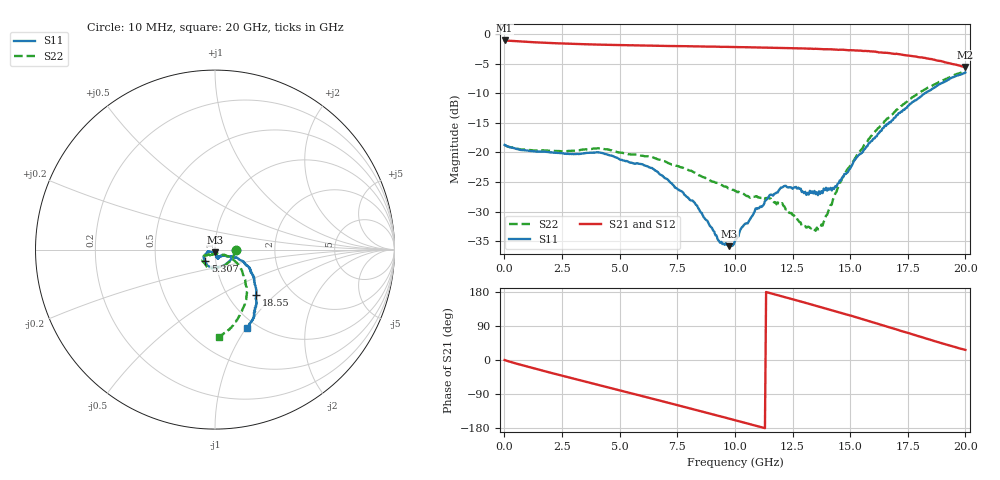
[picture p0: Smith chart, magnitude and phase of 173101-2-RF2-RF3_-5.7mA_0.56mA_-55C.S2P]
!  2-Port S-parameters saved by WinCal
! VAR MeasName=S-Parameters (CALIBRATED_DATA) read from VNA (N5242A)
! VAR MeasDate=2017-7-20 10:24:18
! VAR NAME=173101-2-RF2-RF3_-5.7mA_0.56mA_-55C
! VAR FILENAME=173101-2-RF2-RF3_-5.7mA_0.56mA_-55C.S2P
! VAR DATE=2017-7-20 10:24:18
! VAR PHYS_PORTS=1,2
# Hz S DB R 50
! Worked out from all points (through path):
!   401 points, 10 MHz to 20 GHz, reference 50 ohm
!   highest |S21| = -1.10 dB at 10 MHz (marker M1); lowest = -5.6 dB at 20 GHz (marker M2)
!   group delay of S21, straight-line fit = 45.8 ps
!   lowest |S11| = -35.8 dB at 9.755 GHz (marker M3), VSWR 1.03, Z = 50 - j1.61 ohm
!   |S11| at or under -10 dB: start of sweep to 18.25 GHz
!   |S22| runs from -33.2 to -6.3 dB; largest |S21 - S12| = 0.0092
!   S11 on the Smith chart (normalised r, x): 10 MHz: 1.26, -0.01; 5.307 GHz: 0.89, -0.12; 18.55 GHz: 1.34, -0.77; 20 GHz: 0.90, -1.01
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1e7  -18.75 -2.0  -1.10 -0.0  -1.11 -0.1  -18.75 -1.9
1.559225e9  -19.88 -55.0  -1.46 -26.5  -1.47 -26.6  -19.68 -55.0
3.358325e9  -20.22 -97.9  -1.72 -54.7  -1.73 -54.8  -19.55 -96.1
4.157925e9  -20.05 -113.5  -1.81 -67.1  -1.83 -67.1  -19.32 -111.3
5.30735e9  -21.46 -129.9  -1.91 -84.8  -1.93 -84.8  -20.22 -124.7
6.70665e9  -23.56 -150.4  -2.00 -106.7  -2.00 -106.6  -21.23 -141.5
8.255875e9  -28.53 -163.2  -2.12 -130.9  -2.13 -130.9  -23.42 -151.2
9.355325e9  -35.25 -117.4  -2.18 -148.5  -2.18 -148.4  -25.41 -144.9
9.755125e9  -35.84 -89.0  -2.20 -154.8  -2.20 -154.9  -26.07 -145.6
1.0005e10  -34.94 -84.9  -2.21 -158.8  -2.23 -158.9  -26.49 -144.8
1.090455e10  -29.45 -74.0  -2.28 -173.3  -2.30 -173.3  -27.43 -130.9
1.205398e10  -25.93 -74.3  -2.37 167.9  -2.38 167.9  -28.59 -123.0
1.30035e10  -26.90 -59.4  -2.46 151.9  -2.44 151.9  -32.42 -92.7
1.335332e10  -26.57 -61.4  -2.51 146.0  -2.48 145.9  -32.65 -77.2
1.375312e10  -26.56 -56.3  -2.56 139.0  -2.55 139.0  -32.19 -61.2
1.430285e10  -26.16 -43.3  -2.64 129.6  -2.66 129.6  -27.54 -37.9
1.475262e10  -23.66 -31.1  -2.69 121.7  -2.70 121.5  -23.66 -28.3
1.530235e10  -20.77 -25.2  -2.79 112.0  -2.81 111.7  -20.41 -27.2
1.670165e10  -14.92 -23.8  -3.24 86.3  -3.31 85.9  -14.01 -39.7
1.76012e10  -11.82 -33.9  -3.69 69.9  -3.70 69.7  -10.95 -51.0
1.855072e10  -9.29 -47.9  -4.26 51.9  -4.36 52.0  -8.76 -65.0
2e10  -6.51 -67.7  -5.60 26.6  -5.67 27.2  -6.26 -87.2
